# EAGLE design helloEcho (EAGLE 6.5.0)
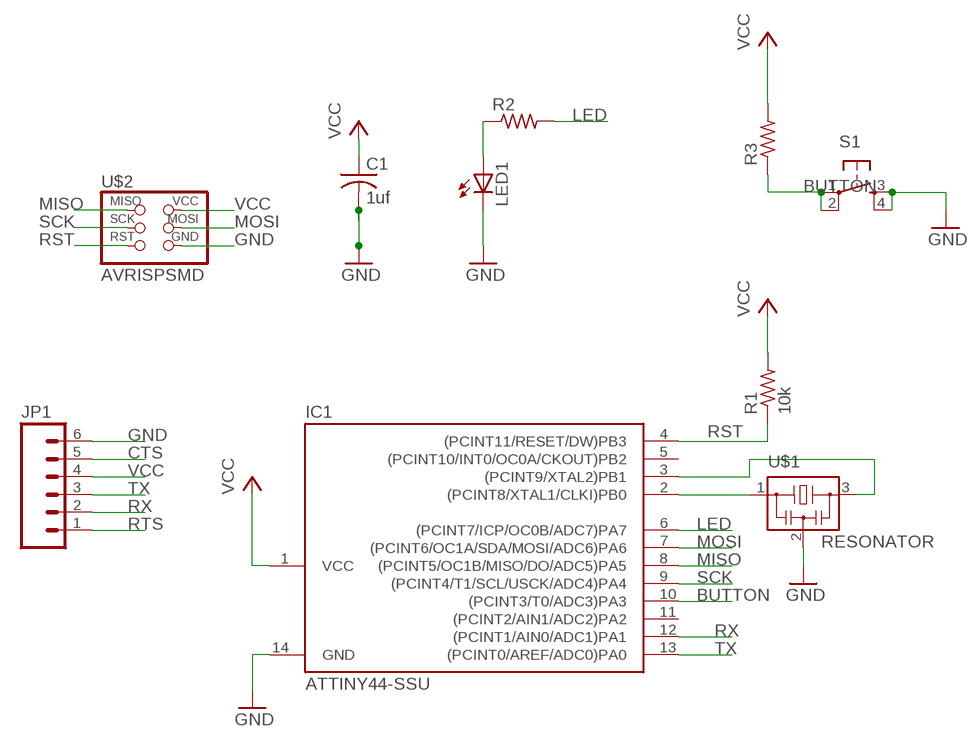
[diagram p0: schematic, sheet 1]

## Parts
C1  1uf  C-USC1206  [C1206]
IC1  ATTINY44-SSU  [SOIC14]
JP1  M06SMD  [1X06-SMD]
LED1  LED1206  [1206]
R1  10k  R-US_R1206  [R1206]
R2  RESISTOR1206  [1206]
R3  RESISTOR1206  [1206]
S1  6MM_SWITCH6MM_SWITCH  [6MM_SWITCH]
U$1  RESONATOR  [EFOBM]
U$2  AVRISPSMD  [2X03SMD]

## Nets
BUTTON: IC1.10((PCINT3/T0/ADC3)PA3) R3.1 S1.1(P) S1.2(P1)
CTS: JP1.5
GND: C1.2 IC1.14(GND) JP1.6 LED1.2(C) S1.3(S) S1.4(S1) U$1.2 U$2.6(GND)
LED: IC1.6((PCINT7/ICP/OC0B/ADC7)PA7) R2.2
MISO: IC1.8((PCINT5/OC1B/MISO/DO/ADC5)PA5) U$2.1(MISO)
MOSI: IC1.7((PCINT6/OC1A/SDA/MOSI/ADC6)PA6) U$2.4(MOSI)
N$1: IC1.2((PCINT8/XTAL1/CLKI)PB0) U$1.1
N$2: IC1.3((PCINT9/XTAL2)PB1) U$1.3
N$3: LED1.1(A) R2.1
RST: IC1.4((PCINT11/RESET/DW)PB3) R1.1 U$2.5(RST)
RTS: JP1.1
RX: IC1.12((PCINT1/AIN0/ADC1)PA1) JP1.2
SCK: IC1.9((PCINT4/T1/SCL/USCK/ADC4)PA4) U$2.3(SCK)
TX: IC1.13((PCINT0/AREF/ADC0)PA0) JP1.3
VCC: C1.1 IC1.1(VCC) JP1.4 R1.2 R3.2 U$2.2(VCC)
Unconnected: IC1.5((PCINT10/INT0/OC0A/CKOUT)PB2) IC1.11((PCINT2/AIN1/ADC2)PA2)

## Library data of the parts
C1 = rcl:C-US: CAPACITOR, American symbol
IC1 = fab:ATTINY44
JP1 = SparkFun:M06: Header 6 Standard 6-pin 0.1" header. Use with straight break away headers (SKU : PRT-00116), right angle break away headers (PRT-00553), swiss pins (PRT-00743), machine pins (PRT-00117), and female headers (PRT-00115). Molex polarized connector foot print use with SKU : PRT-08094 with associated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
LED1 = 01_FAB_Hello:LED
R1 = resistor:R-US_: RESISTOR, American symbol
R2 R3 = 01_FAB_Hello:RESISTOR
S1 = 01_FAB_Hello:6MM_SWITCH: OMRON SWITCH
U$1 = fab:RESONATOR
U$2 = fab:AVRISP

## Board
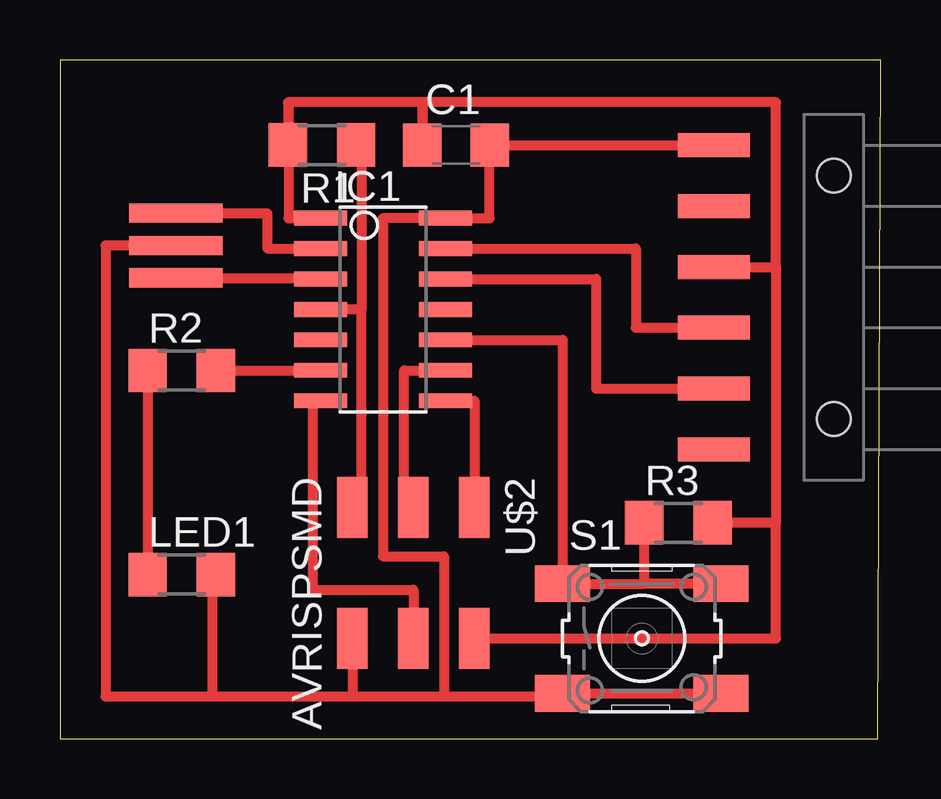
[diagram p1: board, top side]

Size 34.21 x 28.31 mm. Coordinates in mm from the lower left corner, seen from the top.
Outline: 0,0 34.09,0 34.21,28.31 0,28.31 0,0
Copper layers 1: Top 0.035mm
Design rules "ERP-1sided-10mil-16mill": minimum track width 10mil, minimum drill 24mil, track to track 16mil, track to pad 16mil, pad to pad 16mil, via to via 16mil, smd to smd 0mil, copper to edge 16mil, drill to drill 36mil, minimum pad ring 10mil, minimum via ring 8mil, stop-mask expansion 4mil, vias tented up to drill 0mil, thermal gap 10mil

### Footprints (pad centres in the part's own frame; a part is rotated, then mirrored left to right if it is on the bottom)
C1206 = smd 1.6 x 1.8: 1 -1.4,0; 2 1.4,0
SOIC14 = smd 0.61 x 2.21: 1 -3.81,-2.603; 2 -2.54,-2.603; 3 -1.27,-2.603; 4 0,-2.603; 5 1.27,-2.603; 6 2.54,-2.603; 7 3.81,-2.603; 8 3.81,2.603; 9 2.54,2.603; 10 1.27,2.603; 11 0,2.603; 12 -1.27,2.603; 13 -2.54,2.603; 14 -3.81,2.603
1X06-SMD = smd 1 x 3: 1 -6.35,5; 2 -3.81,5; 3 -1.27,5; 4 1.27,5; 5 3.81,5; 6 6.35,5 | hole 1.4: -5.08,0; 5.08,0
1206 = smd 1.6 x 1.803: 1 -1.422,0; 2 1.422,0
R1206 = smd 1.6 x 1.803: 1 -1.422,0; 2 1.422,0
6MM_SWITCH = smd 2.286 x 1.524: 1 -3.302,2.286; 2 3.302,2.286; 3 -3.302,-2.286; 4 3.302,-2.286
EFOBM = smd 0.8 x 3.9: 1 -1.35,0; 2 0,0; 3 1.35,0
2X03SMD = smd 2.54 x 1.27: 1 -2.54,2.54; 2 2.92,2.54; 3 -2.54,0; 4 2.92,0; 5 -2.54,-2.54; 6 2.92,-2.54

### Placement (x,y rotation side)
C1  16.51,24.77 0 top
IC1  13.46,17.91 270 top
JP1  32.26,18.41 90 top
LED1  5.08,6.86 0 top
R1  10.92,24.77 180 top
R2  5.08,15.37 0 top
R3  25.78,9.02 0 top
S1  24.26,4.19 0 top
U$1  4.83,20.57 270 top
U$2  14.73,7.11 270 top

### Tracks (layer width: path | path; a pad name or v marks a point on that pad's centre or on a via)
BUTTON
  Top 0.406: IC1.10 20.95,16.64 S1.1 24.36,6.48 | 24.36,6.48 R3.1 | S1.2 24.36,6.48
GND
  Top 0.406: JP1.6 C1.2 17.91,21.72 IC1.14 13.46,21.72 13.46,7.62 16,7.62 16,1.78 | U$1.2 1.91,20.57 1.91,1.78 6.35,1.78 | 6.35,1.78 12.19,1.78 | 12.19,1.78 16,1.78 | 16,1.78 20.95,1.78 S1.3 S1.4 | U$2.6 12.19,1.78 | LED1.2 6.35,6.86 6.35,1.78
LED
  Top 0.406: R2.2 IC1.6
MISO
  Top 0.406: IC1.8 17.27,14.1 U$2.1
MOSI
  Top 0.406: IC1.7 10.54,14.1 10.54,6.22 14.73,6.22 U$2.4
N$1
  Top 0.406: U$1.1 8.64,21.92 8.64,20.45 IC1.2 11.11,20.45
N$2
  Top 0.406: U$1.3 10.6,19.22 IC1.3
N$3
  Top 0.406: R2.1 LED1.1
N$12
  Top 0.406: 5.08,20.7 5.08,20.45
N$15
  Top 0.406: 12.19,24.13 12.32,24.13
N$18
  Top 0.406: 27.43,14.61 27.43,14.48
RST
  Top 0.406: U$2.5 12.57,9.65 12.57,17.91 | 12.57,17.91 IC1.4 | R1.1 12.57,24.77 12.57,17.91
RX
  Top 0.406: IC1.12 22.35,19.18 22.35,14.61 JP1.2
SCK
  Top 0.406: U$2.3 14.35,9.65 14.35,15.37 IC1.9
TX
  Top 0.406: IC1.13 24,20.45 24,17.14 JP1.3
VCC
  Top 0.406: 11.18,21.72 IC1.1 | IC1.1 10.54,21.72 | U$2.2 29.84,4.19 29.84,9.02 | 29.84,9.02 R3.2 | 29.84,19.68 29.84,9.02 | JP1.4 29.84,19.68 | 29.84,19.68 29.84,26.54 15.11,26.54 | 15.11,26.54 | 15.11,26.54 C1.1 15.11,26.54 | 15.11,26.54 9.53,26.54 | 9.53,26.54 9.53,21.72 IC1.1 | 9.53,26.54 9.5,26.54 R1.2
